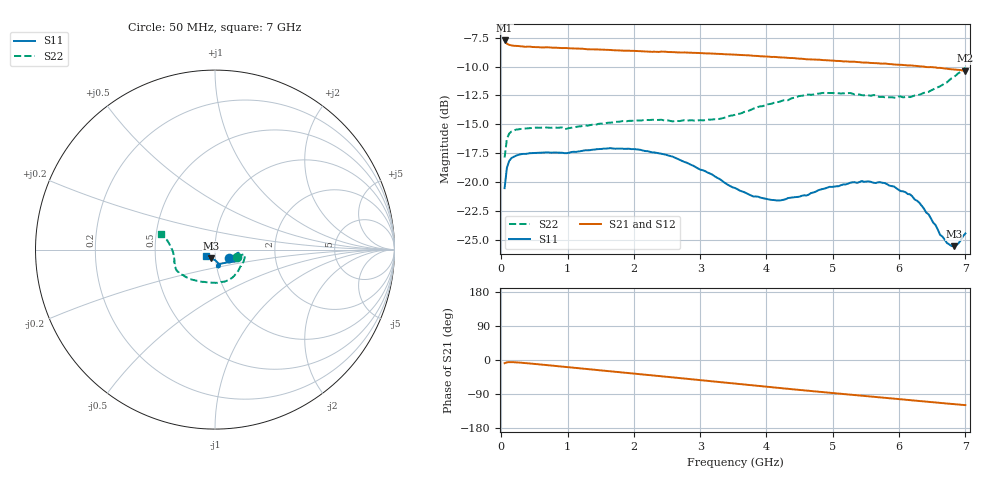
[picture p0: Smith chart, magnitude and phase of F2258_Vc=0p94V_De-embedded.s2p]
! Integrated Device Technology
! Corporate Headquarters
! 6024 Silver Creek Valley Road
! San Jose, CA 95138  USA
! Phone:  1-408-284-8200
! Toll Free:  1-800-223-1366
! Webpage:  http://www.idt.com/
! Timing and RF Division
! 515 Groton Road, Suite 102
! Westford, MA 01886-6024
! Device:  F2258
! Description: Voltage Variable RF Attenuator
! Frequency:  50.0 -  6000.00 MHz
! Package:  3x3 mm Thin QFN Plastic Package: 16 pin
! Ports:  2 RF, 2 DC
!  Pin  1  = NC
!  Pin  2  = NC
!  Pin  3  = RF2  = Port 2
!  Pin  4  = GND
!  Pin  5  = Vdd
!  Pin  6  = NC
!  Pin  7  = VCTRL
!  Pin  8  = NC
!  Pin  9  = GND
!  Pin 10  = RF1  = Port 1
!  Pin 11  = NC
!  Pin 12  = NC
!  Pin 13  = NC
!  Pin 14  = NC
!  Pin 15  = NC
!  Pin 16  = NC
! Vcntrl:  0.940 Volts
! Vdd:  +3.300 Volts
! Current:  1.152 mA
! Data:  The device was measured on a the F2258 evaluation board which has
!  individual transmission lines to the RF pins.  Data was collected
!  using a calibrated network analyzer.  The evaluation board was
!  de-embedded using a TRL calibration technique.
!  The reference plane is the edge of the package pin.
! Misc:  SN 10
!  Action Tracker AT0285
! Date Measured:  2014-12-10
! Date:  2016-01-13  MJV
! Note:
!  Integrated Device Technology supplies this data as a sample of measured
!  data at the package pin for this product.  Your particular data for this
!  product may vary.
!  Data was taken at 25 degrees C.
!  Integrated Device Technology reserves the right to change this data at anytime.
!Freq_(GHz)  S11M_(dB)  S11P_(deg)  S21M_(dB)  S21P_(deg)  S12M_(dB)  S12P_(deg)  S22M_(dB)  S22P_(deg)
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# GHz S dB R 50
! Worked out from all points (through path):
!   201 points, 50 MHz to 7 GHz, reference 50 ohm
!   highest |S21| = -7.74 dB at 50 MHz (marker M1); lowest = -10.4 dB at 7 GHz (marker M2)
!   group delay of S21, straight-line fit = 46.7 ps
!   lowest |S11| = -25.5 dB at 6.826 GHz (marker M3), VSWR 1.11, Z = 47.6 - j4.59 ohm
!   |S11| at or under -10 dB: start of sweep to end of sweep
!   |S22| runs from -17.9 to -10.1 dB; largest |S21 - S12| = 0.0023
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0.05  -20.52 -31.1  -7.74 -8.3  -7.74 -8.3  -17.87 -19.2
0.08475  -18.75 -14.9  -8.03 -6.2  -8.02 -6.2  -16.25 -10.7
0.1195  -18.16 -10.3  -8.12 -5.6  -8.11 -5.6  -15.79 -9.3
0.22375  -17.71 -7.7  -8.21 -6.2  -8.21 -6.2  -15.46 -10.2
0.9535  -17.49 -17.9  -8.39 -18.1  -8.39 -18.1  -15.42 -33.1
1.2315  -17.28 -20.7  -8.46 -22.9  -8.45 -22.9  -15.13 -41.7
1.9265  -17.11 -26.0  -8.63 -34.6  -8.64 -34.6  -14.70 -60.6
2.37825  -17.51 -29.2  -8.73 -42.3  -8.73 -42.3  -14.61 -73.2
3.0385  -18.97 -37.9  -8.84 -53.7  -8.87 -53.7  -14.66 -95.5
3.525  -20.51 -50.9  -8.97 -62.3  -9.00 -62.3  -14.17 -115.0
3.803  -21.24 -61.8  -9.07 -67.1  -9.09 -67.1  -13.64 -125.5
4.1505  -21.58 -73.2  -9.18 -73.1  -9.22 -73.1  -13.07 -135.9
4.7065  -20.89 -83.1  -9.39 -82.4  -9.41 -82.4  -12.42 -148.6
5.43625  -19.90 -79.1  -9.65 -94.2  -9.67 -94.1  -12.47 -160.4
5.85325  -20.30 -74.3  -9.78 -100.8  -9.82 -100.8  -12.66 -168.9
6.166  -21.05 -74.0  -9.90 -105.9  -9.93 -105.9  -12.64 -176.3
6.305  -21.78 -75.5  -9.98 -108.2  -10.00 -108.1  -12.44 -180.0
6.54825  -23.70 -83.9  -10.07 -112.1  -10.12 -112.0  -11.88 173.7
6.61775  -24.55 -88.8  -10.11 -113.1  -10.15 -113.1  -11.70 171.8
6.722  -25.26 -99.7  -10.18 -114.8  -10.22 -114.8  -11.37 169.1
6.82625  -25.54 -114.6  -10.25 -116.4  -10.28 -116.4  -10.91 167.2
7  -24.44 -142.2  -10.37 -119.0  -10.39 -119.0  -10.09 163.8
